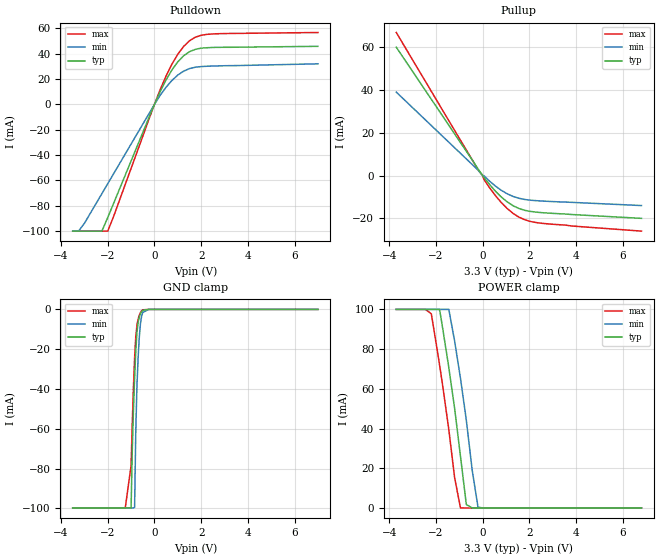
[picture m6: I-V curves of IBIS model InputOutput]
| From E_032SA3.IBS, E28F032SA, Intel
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|***********************Input Output Model***********************
[Model]   InputOutput
Model_type   I/O
|   for DQ[15:0]
Vinl = 0.8V
Vinh = 2.0V
| Variable   typ   min   max
C_comp   9.61p   NA   11.6p
[Voltage Range]   3.3V   3.0V   3.6V
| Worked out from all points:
|   slope of the pulldown table from 0 to 0.495 V, typ, clamps not added: 25.8 ohm
|   slope of the pullup table from 0 to 0.495 V, typ, clamps not added: 74.3 ohm
|   GND clamp passes 1 mA (typ) near -0.54 V on its own axis
|   POWER clamp passes 1 mA (typ) near -0.59 V on its own axis
[Pulldown]
| [Pullup] and [Pulldown] IV curves include only the current through
| the channels of output driver transistors when outputs are enabled
| with OE# = VIL.  Although the output driver transistors have np and
| pn diodes inherently created by CMOS IC fabrication between the
| drain and bulk of n-channel and p-channel CMOS transistors,
| the current through these junction diodes is not included in
| [Pullup] or [Pulldown].  Instead that drain/bulk diode current is
| included in the [POWER_clamp] or [GND_clamp] sections, which are
| not dependent on the state of OE# or output data value.
|Voltage  I(typ)   I(min)   I(max)
-3.5V     -100mA     -100mA     -100mA
-3.25V    -100mA     -100mA     -100mA
-3V       -100mA     -93.88mA   -100mA
-2.25V    -100mA     -70.41mA   -100mA
-2V       -89.32mA   -62.58mA   -100mA
250mV     10.31mA    7.306mA    11.9mA
750mV     27.19mA    18.89mA    31.78mA
1V        33.56mA    23.13mA    39.59mA
1.5V      41.57mA    28.24mA    50.16mA
2V        44.38mA    29.82mA    54.53mA
2.5V      44.92mA    30.26mA    55.58mA
7V        45.8mA     32mA       56.7mA
[GND_clamp]
| [POWER_clamp] and [GND_clamp] IV curves describe ESD protection
| circuits PLUS some np and pn diodes which exist between the
| drain and bulk of n-channel and p-channel CMOS transistors.
| These drain/bulk diodes are inherent in CMOS IC fabrication,
| and are visible on the node of the I/O pin at all times.
| Even the drain/bulk diodes of output driver [Pullup] and [Powerdown]
| transistors are included in [POWER_clamp] or [GND_clamp], because
| these diodes contribute to I/O pin current even when the
| chip outputs are tristated by OE# = VIH.
| For example, when V forced on the I/O pin is large, we are
| forward biasing the pn diode at the drain/bulk interface in the
| p-channel pullup transistor.  Similarly, when V forced on the
| I/O pin is sufficiently negative with respect to the substrate
| ground, we are forward biasing the np diode at the drain/bulk
| interface in the n-channel pulldown transistor.  The effects
| of these diodes are included in [POWER_clamp] or [GND_clamp].
|Voltage  I(typ)   I(min)   I(max)
-3.5V     -99.84mA   -99.84mA   -99.85mA
-1.25V    -99.84mA   -99.84mA   -99.85mA
-1V       -99.84mA   -99.84mA   -78.52mA
-950mV    -71.19mA   -99.84mA   -57.54mA
-900mV    -50.96mA   -99.84mA   -39.26mA
-850mV    -34.78mA   -99.62mA   -24.43mA
-800mV    -21.1mA    -61.65mA   -13.82mA
-750mV    -11.75mA   -38.54mA   -8.01mA
-650mV    -3.891mA   -14.15mA   -2.999mA
-600mV    -2.235mA   -7.162mA   -1.606mA
-500mV    -459.6uA   -1.565mA   -211.6uA
7V        0A         0A         0A
[Pullup]
| (Voltages for [Pullup] and [POWER_clamp] are specified with
| negative respect to Vcc.  Reference the IBIS documentation
| for more information regarding Vtable = Vcc - Voutput.
| This method keeps -Vds constant for the values in all three
| columns across a line of the table.
| [Pullup] and [Pulldown] IV curves include only the current through
| the channels of output driver transistors when outputs are enabled
| with OE# = VIL.  Although the output driver transistors have np and
| pn diodes inherently created by CMOS IC fabrication between the
| drain and bulk of n-channel and p-channel CMOS transistors,
| the current through these junction diodes is not included in
| [Pullup] or [Pulldown].  Instead that drain/bulk diode current is
| included in the [POWER_clamp] or [GND_clamp] sections, which are
| not dependent on the state of OE# or output data value.
|Voltage  I(typ)   I(min)   I(max)
-3.7V     59.95mA    38.98mA    66.81mA
-200mV    3.127mA    2.572mA    2.671mA
0V        0A         0A         0A
50mV      -744.5uA   -264.5nA   -1.741mA
550mV     -7.345mA   -4.949mA   -9.428mA
800mV     -10.05mA   -6.905mA   -12.64mA
1.3V      -14.07mA   -9.734mA   -17.65mA
1.8V      -16.22mA   -11.16mA   -20.63mA
2.3V      -17.09mA   -11.72mA   -21.96mA
6.8V      -19.98mA   -14mA      -25.94mA
[POWER_clamp]
| (Voltages for [Pullup] and [POWER_clamp] are specified with
| negative respect to Vcc.  Reference the IBIS documentation
| for more information regarding Vtable = Vcc - Voutput.
| This method keeps -Vds constant for the values in all three
| columns across a line of the table.
| [POWER_clamp] and [GND_clamp] IV curves describe ESD protection
| circuits PLUS some np and pn diodes which exist between the
| drain and bulk of n-channel and p-channel CMOS transistors.
| These drain/bulk diodes are inherent in CMOS IC fabrication,
| and are visible on the node of the I/O pin at all times.
| Even the drain/bulk diodes of output driver [Pullup] and [Powerdown]
| transistors are included in [POWER_clamp] or [GND_clamp], because
| these diodes contribute to I/O pin current even when the
| chip outputs are tristated by OE# = VIH.
| For example, when V forced on the I/O pin is large, we are
| forward biasing the pn diode at the drain/bulk interface in the
| p-channel pullup transistor.  Similarly, when V forced on the
| I/O pin is sufficiently negative with respect to the substrate
| ground, we are forward biasing the np diode at the drain/bulk
| interface in the n-channel pulldown transistor.  The effects
| of these diodes are included in [POWER_clamp] or [GND_clamp].
|Voltage  I(typ)   I(min)   I(max)
-3.7V     100mA      100mA      100mA
-2.45V    100mA      100mA      100mA
-2.2V     100mA      100mA      97.77mA
-1.85V    100mA      100mA      72.28mA
-1.7V     89.53mA    100mA      60.56mA
-1.45V    70.71mA    100mA      39.43mA
-1.2V     50.02mA    83.94mA    15.16mA
-950mV    26mA       65.25mA    36.7uA
-700mV    1.736mA    44.18mA    0A
-450mV    0A         19.11mA    0A
-200mV    0A         387.4uA    0A
6.8V      0A         0A         0A
[Ramp]
| The DQ Ramp information is not provided at this time for the
| device but will be available in the future.  The table below
| is for the compatibility with some IBIS parsers.
| Variable   typ   min   max
 dV/dt_r   0V/0ns   0V/0ns   0V/0ns
 dV/dt_f   0V/0ns   0V/0ns   0V/0ns
